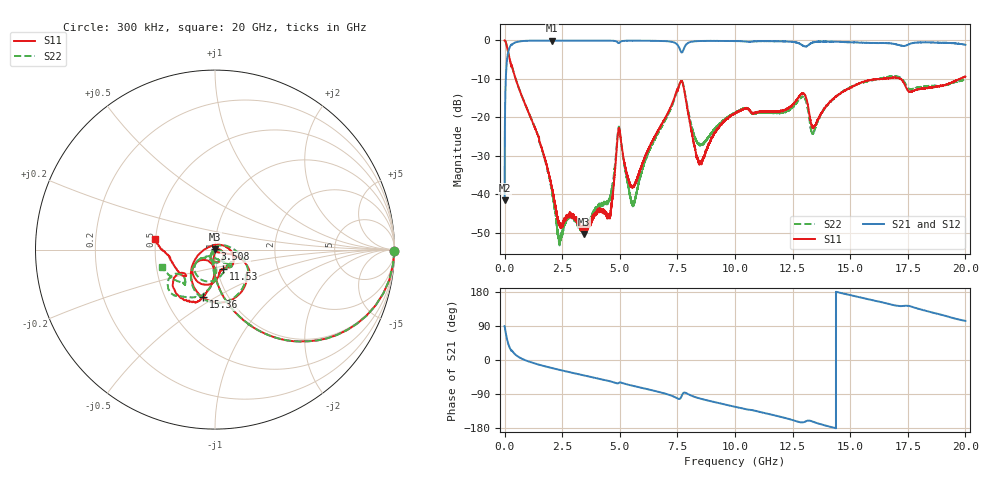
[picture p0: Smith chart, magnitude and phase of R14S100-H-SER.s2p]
!{R14S100}
!Johanson Technology Inc.
!www.johansontechnology.com
!Test Board Conditions:
!Substrate Type  RO4350B
!Substrate Thickness  20 mil
!Substrate Dk  3.66
!TL Type: GCPW
!TL Trace Width  36 mil
!TL Gap  12 mil
!Electrode orientation  Horizontal
!DUT TOPOLOGY	SERIES
!Mounting Pad LxW  26x36 mil
! Created Wed Nov 25 17:33:21 2020
! 2 Port Network Data from SP1.SP block
! freq  magS11  angS11  magS21  angS21  magS12  angS12  magS22  angS22
# khz S ma R 50
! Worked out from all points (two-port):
!   20001 points, 300 kHz to 20 GHz, reference 50 ohm
!   highest |S21| = -0.01 dB at 2.071 GHz (marker M1); lowest = -41.5 dB at 300 kHz (marker M2)
!   |S21| within 3 dB of the highest: 156.3 MHz to 7.663 GHz (7.506 GHz wide, 192 % of centre); 7.719 GHz to end of sweep
!   lowest |S11| = -50.4 dB at 3.429 GHz (marker M3), VSWR 1.01, Z = 50 + j0.303 ohm
!   |S11| at or under -10 dB: 480.1 MHz to 16.35 GHz (15.86 GHz wide, 189 % of centre); 16.35951 GHz to 16.42217 GHz (62.66 MHz wide, 0.382 % of centre); 17.18 GHz to 19.76 GHz (2.58 GHz wide, 14 % of centre)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
!   |S22| runs from -53.5 to 0.0 dB; largest |S21 - S12| = 0.02
!   S11 on the Smith chart (normalised r, x): 300 kHz: open; 3.508 GHz: 1.00, +0.01; 11.53 GHz: 1.07, -0.24; 15.36 GHz: 0.76, -0.44; 20 GHz: 0.50, +0.07
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300  1 -0.4  0.008374 89.6  0.008358 89.3  0.9998 -0.4
111300  0.811 -36.8  0.581 53.1  0.5818 52.9  0.812 -36.8
237300  0.5421 -59.5  0.8355 30.3  0.8363 30.2  0.5433 -59.4
708300  0.2033 -84.7  0.9761 4.7  0.9769 4.7  0.2031 -85.1
2071300  0.01139 -89.4  0.9984 -21.5  0.9977 -21.5  0.01026 -125.9
2381300  0.004119 -34.2  0.997 -26.0  0.9974 -26.0  0.00245 151.1
3334300  0.003519 70.2  0.9961 -39.2  0.996 -39.2  0.003596 17.8
3429300  0.003033 87.1  0.9948 -40.4  0.9959 -40.5  0.003206 1.0
3508300  0.003348 96.3  0.9963 -41.5  0.9959 -41.5  0.003793 -12.4
4546300  0.005002 84.6  0.9926 -55.8  0.9929 -55.8  0.008584 -34.3
4956300  0.07214 -68.1  0.9216 -60.4  0.9216 -60.3  0.07521 -66.3
5569300  0.01263 -86.4  0.9922 -68.1  0.9933 -68.2  0.007385 139.8
6667300  0.06769 -19.3  0.9885 -83.9  0.9872 -83.9  0.06288 21.1
7660300  0.2965 -75.8  0.7089 -98.3  0.7095 -98.3  0.2974 -78.9
8476300  0.02453 103.1  0.9822 -101.6  0.9832 -101.5  0.0439 -111.1
1.00003e7  0.1128 -23.2  0.9814 -123.4  0.9806 -123.5  0.1149 -46.0
1.15283e7  0.118 -66.8  0.9788 -143.4  0.9779 -143.3  0.1145 -40.6
1.29583e7  0.2051 -114.2  0.853 -164.4  0.8543 -164.5  0.1841 -114.0
1.33343e7  0.0779 -130.7  0.9313 -161.8  0.9316 -161.8  0.06354 -128.6
1.53623e7  0.2746 -104.2  0.9395 166.2  0.9443 166.0  0.2745 -108.2
1.66673e7  0.3194 -117.3  0.9205 148.1  0.9123 147.8  0.3385 -130.3
2e7  0.338 169.9  0.8779 103.2  0.8756 103.4  0.3082 -162.3
